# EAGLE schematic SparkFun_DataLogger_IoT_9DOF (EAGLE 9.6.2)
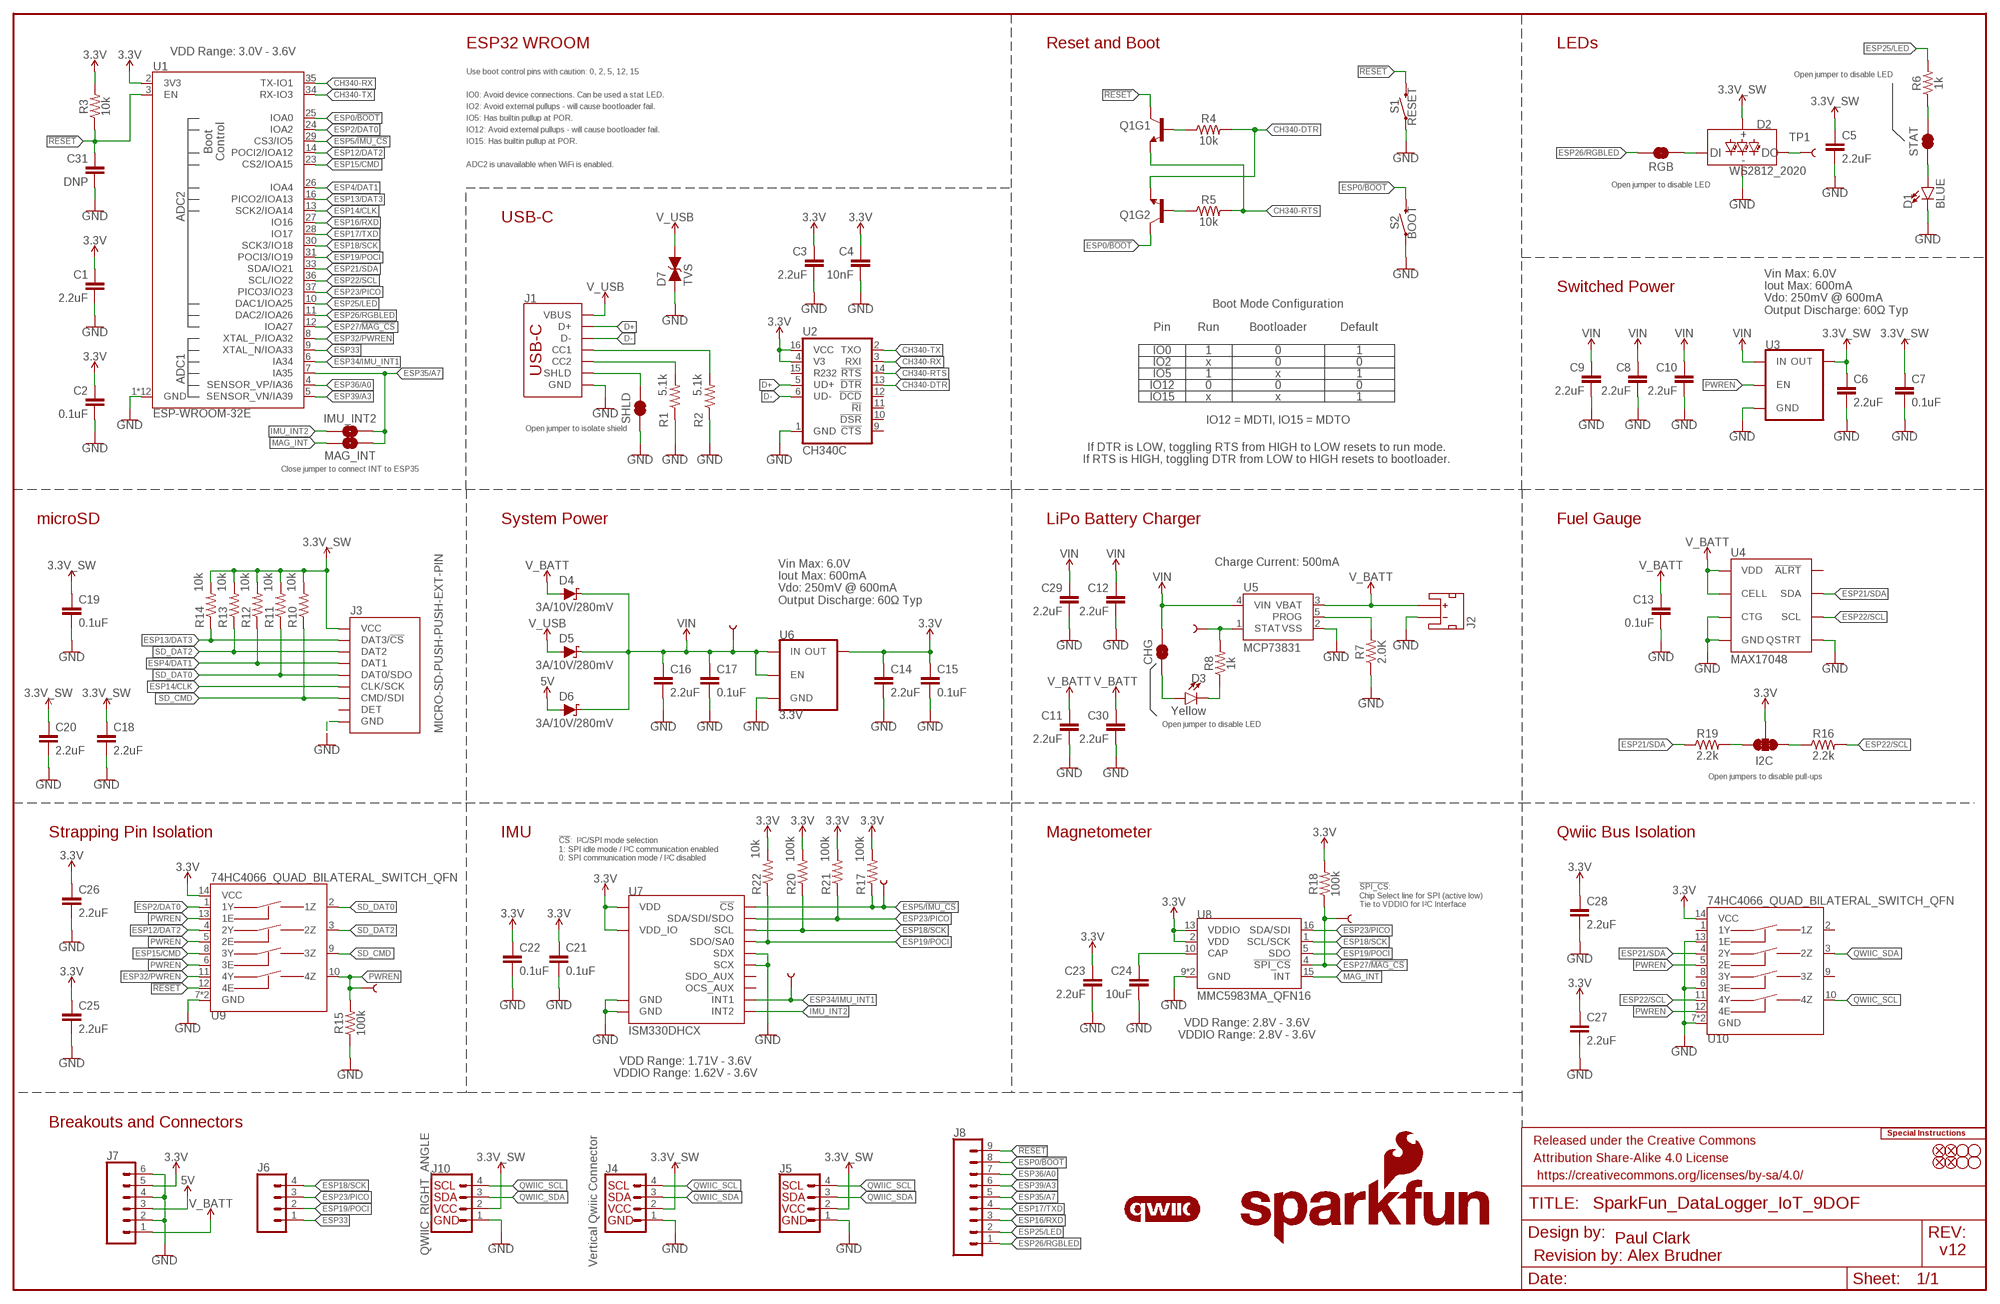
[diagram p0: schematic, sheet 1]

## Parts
C1  2.2uF  2.2UF-0402_TIGHT-10V-10%-X5R  [0402-TIGHT]
C2  0.1uF  0.1UF-0402T-6.3V-10%-X7R  [0402-TIGHT]
C3  2.2uF  2.2UF-0402_TIGHT-10V-10%-X5R  [0402-TIGHT]
C4  10nF  10NF-0402T-25V-10%-X7R-WE  [0402-TIGHT]
C5  2.2uF  2.2UF-0402_TIGHT-10V-10%-X5R  [0402-TIGHT]
C6  2.2uF  2.2UF-0402_TIGHT-10V-10%-X5R  [0402-TIGHT]
C7  0.1uF  0.1UF-0402T-6.3V-10%-X7R  [0402-TIGHT]
C8  2.2uF  2.2UF-0402_TIGHT-10V-10%-X5R  [0402-TIGHT]
C9  2.2uF  2.2UF-0402_TIGHT-10V-10%-X5R  [0402-TIGHT]
C10  2.2uF  2.2UF-0402_TIGHT-10V-10%-X5R  [0402-TIGHT]
C11  2.2uF  2.2UF-0402_TIGHT-10V-10%-X5R  [0402-TIGHT]
C12  2.2uF  2.2UF-0402_TIGHT-10V-10%-X5R  [0402-TIGHT]
C13  0.1uF  0.1UF-0402T-6.3V-10%-X7R  [0402-TIGHT]
C14  2.2uF  2.2UF-0402_TIGHT-10V-10%-X5R  [0402-TIGHT]
C15  0.1uF  0.1UF-0402T-6.3V-10%-X7R  [0402-TIGHT]
C16  2.2uF  2.2UF-0402_TIGHT-10V-10%-X5R  [0402-TIGHT]
C17  0.1uF  0.1UF-0402T-6.3V-10%-X7R  [0402-TIGHT]
C18  2.2uF  2.2UF-0402_TIGHT-10V-10%-X5R  [0402-TIGHT]
C19  0.1uF  0.1UF-0402T-6.3V-10%-X7R  [0402-TIGHT]
C20  2.2uF  2.2UF-0402_TIGHT-10V-10%-X5R  [0402-TIGHT]
C21  0.1uF  0.1UF-0402T-6.3V-10%-X7R  [0402-TIGHT]
C22  0.1uF  0.1UF-0402T-6.3V-10%-X7R  [0402-TIGHT]
C23  2.2uF  2.2UF-0402_TIGHT-10V-10%-X5R  [0402-TIGHT]
C24  10uF  10UF-0402T-6.3V-20%  [0402-TIGHT]
C25  2.2uF  2.2UF-0402_TIGHT-10V-10%-X5R  [0402-TIGHT]
C26  2.2uF  2.2UF-0402_TIGHT-10V-10%-X5R  [0402-TIGHT]
C27  2.2uF  2.2UF-0402_TIGHT-10V-10%-X5R  [0402-TIGHT]
C28  2.2uF  2.2UF-0402_TIGHT-10V-10%-X5R  [0402-TIGHT]
C29  2.2uF  2.2UF-0402_TIGHT-10V-10%-X5R  [0402-TIGHT]
C30  2.2uF  2.2UF-0402_TIGHT-10V-10%-X5R  [0402-TIGHT]
C31  DNP  DNP-0402-TIGHT_NO_CREAM  [0402-TIGHT_NO_CREAM]
CHG  JUMPER-SMT_2_NC_TRACE_SILK  [SMT-JUMPER_2_NC_TRACE_SILK]
D1  BLUE  LED-BLUE0603  [LED-0603]
D2  WS2812_2020  [WS2812-2020]
D3  Yellow  LED-YELLOW0603  [LED-0603]
D4  3A/10V/280mV  DIODE-SCHOTTKY-BAT60A  [SOD-323]
D5  3A/10V/280mV  DIODE-SCHOTTKY-BAT60A  [SOD-323]
D6  3A/10V/280mV  DIODE-SCHOTTKY-BAT60A  [SOD-323]
D7  TVS  DIODE_TVS  [0603]
FD1  FIDUCIAL1X2  [FIDUCIAL-1X2]
FD2  FIDUCIAL1X2  [FIDUCIAL-1X2]
FD3  FIDUCIAL1X2  [FIDUCIAL-1X2]
FD4  FIDUCIAL1X2  [FIDUCIAL-1X2]
FRAME1  FRAME-LEDGER  [CREATIVE_COMMONS]
H1  STAND-OFFTIGHT  [STAND-OFF-TIGHT]
H2  STAND-OFFTIGHT  [STAND-OFF-TIGHT]
H3  STAND-OFFTIGHT  [STAND-OFF-TIGHT]
H4  STAND-OFFTIGHT  [STAND-OFF-TIGHT]
I2C  JUMPER-SMT_3_2-NC_TRACE_SILK  [SMT-JUMPER_3_2-NC_TRACE_SILK]
IMU_!CS!  TEST-POINT3X5  [PAD.03X.05]
IMU_INT1  TEST-POINT3X5  [PAD.03X.05]
IMU_INT2  JUMPER-SMT_2_NO_SILK  [SMT-JUMPER_2_NO_SILK]
J1  USB_C_4-LAYER_PADS  [USB-C-16P_4LAYER-PADS]
J2  JST_2MM_MALE  [JST-2-SMD]
J3  MICRO-SD-PUSH-PUSH-EXT-PIN  [MICROSD-EXTERNALPIN]
J4  Vertical Qwiic Connector  QWIIC_CONNECTOR  [JST04_1MM_VERT]
J5  I2C_STANDARD_NO_SILK  [1X04_NO_SILK]
J6  CONN_041X04_NO_SILK_NO_POP  [1X04_NO_SILK]
J7  CONN_06NO_SILK_NO_POP  [1X06_NO_SILK]
J8  CONN_09NO_SILK  [1X09_NO_SILK]
J10  QWIIC_RIGHT_ANGLE  QWIIC_CONNECTORJS-1MM  [JST04_1MM_RA]
LOGO1  SPECIAL_INSTRUCTIONS-ORDERING  [ORDERING_INSTRUCTIONS]
LOGO3  QWIIC_LOGO_6MM  [QWIIC_6MM]
LOGO5  SFE_LOGO_NAME.2_INCH  [SFE_LOGO_NAME_.2]
LOGO6  SFE_LOGO_FLAME.2_INCH  [SFE_LOGO_FLAME_.2]
MAG_!CS!  TEST-POINT3X5  [PAD.03X.05]
MAG_INT  JUMPER-SMT_2_NO_SILK  [SMT-JUMPER_2_NO_SILK]
PWREN  TEST-POINT3X5  [PAD.03X.05]
Q1  TRANS_NPN_DUAL-MBT3904DW1T1  [SC70-6]
R1  5.1k  5.1KOHM-0402T-1/16W-1%  [0402-TIGHT]
R2  5.1k  5.1KOHM-0402T-1/16W-1%  [0402-TIGHT]
R3  10k  10KOHM-0402T-1/16W-1%  [0402-TIGHT]
R4  10k  10KOHM-0402T-1/16W-1%  [0402-TIGHT]
R5  10k  10KOHM-0402T-1/16W-1%  [0402-TIGHT]
R6  1k  1KOHM-0402T-1/16W-1%  [0402-TIGHT]
R7  2.0K  2.0KOHM-0402T-1/16W-1%  [0402-TIGHT]
R8  1k  1KOHM-0402T-1/16W-1%  [0402-TIGHT]
R10  10k  10KOHM-0402T-1/16W-1%  [0402-TIGHT]
R11  10k  10KOHM-0402T-1/16W-1%  [0402-TIGHT]
R12  10k  10KOHM-0402T-1/16W-1%  [0402-TIGHT]
R13  10k  10KOHM-0402T-1/16W-1%  [0402-TIGHT]
R14  10k  10KOHM-0402T-1/16W-1%  [0402-TIGHT]
R15  100k  100KOHM-0402T-1/16W-1%  [0402-TIGHT]
R16  2.2k  2.2KOHM-0402T-1/16W-1%  [0402-TIGHT]
R17  100k  100KOHM-0402T-1/16W-1%  [0402-TIGHT]
R18  100k  100KOHM-0402T-1/16W-1%  [0402-TIGHT]
R19  2.2k  2.2KOHM-0402T-1/16W-1%  [0402-TIGHT]
R20  100k  100KOHM-0402T-1/16W-1%  [0402-TIGHT]
R21  100k  100KOHM-0402T-1/16W-1%  [0402-TIGHT]
R22  10k  10KOHM-0402T-1/16W-1%  [0402-TIGHT]
RGB  JUMPER-SMT_2_NC_TRACE_SILK  [SMT-JUMPER_2_NC_TRACE_SILK]
S1  RESET  MOMENTARY-SWITCH-SPST-SMD-RIGHT-ANGLE  [TACTILE_SWITCH_SMD_RIGHT_ANGLE]
S2  BOOT  MOMENTARY-SWITCH-SPST-SMD-RIGHT-ANGLE  [TACTILE_SWITCH_SMD_RIGHT_ANGLE]
SHLD  JUMPER-SMT_2_NC_TRACE_SILK  [SMT-JUMPER_2_NC_TRACE_SILK]
STAT  JUMPER-SMT_2_NC_TRACE_SILK  [SMT-JUMPER_2_NC_TRACE_SILK]
TP1  TEST-POINT3X5  [PAD.03X.05]
U1  ESP-WROOM-32E  ESP-WROOM-3232D-NARROW  [ESP-WROOM-32D-NARROW]
U2  CH340C  [SO016]
U3  3.3V  V_REG_AP2112K-3.3V  [SOT23-5]
U4  MAX17048  MAX17048DFN8  [DFN-8]
U5  MCP73831  [SOT23-5]
U6  3.3V  V_REG_AP2112K-3.3V  [SOT23-5]
U7  ISM330DHCX  [LGA-14L]
U8  MMC5983MA_QFN16  [LGA-16-3X3MM-4X4PINS]
U9  74HC4066_QUAD_BILATERAL_SWITCH_QFN  [14-QFN]
U10  74HC4066_QUAD_BILATERAL_SWITCH_QFN  [14-QFN]
VIN  TEST-POINT3X5  [PAD.03X.05]
VIN1  TEST-POINT3X5  [PAD.03X.05]

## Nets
3.3V: C1.1 C2.1 C3.1 C4.1 C14.1 C15.1 C21.1 C22.1 C23.1 C25.1 C26.1 C27.1 C28.1 I2C.2 J7.5 R3.2 R17.2 R18.2 R20.2 R21.2 R22.2 U1.2(3V3) U2.4(V3) U2.16(VCC) U6.5(OUT) U7.P5(VDD_IO) U7.P8(VDD) U8.2(VDD) U8.13(VDDIO) U9.14(VCC) U10.14(VCC)
3.3V_SW: C5.1 C6.1 C7.1 C18.1 C19.1 C20.1 D2.VCC J3.4(VCC) J4.2 J5.2 J10.2 R10.2 R11.2 R12.2 R13.2 R14.2 U3.5(OUT)
5V: D6.A J7.3
!RESET!: C31.1 J8.9 Q1.3(C) R3.1 S1.2 U1.3(EN) U9.12(4E)
CAP: C24.1 U8.10(CAP)
CH340-DTR: Q1.1(E) R4.2 U2.13(!DTR)
CH340-RTS: Q1.4(E) R5.2 U2.14(!RTS)
CH340-RX: U1.35(TX-IO1) U2.3(RXI)
CH340-TX: U1.34(RX-IO3) U2.2(TXO)
D+: J1.A6(D+) J1.B6(D+) U2.5(UD+)
D-: J1.A7(D-) J1.B7(D-) U2.6(UD-)
ESP0/!BOOT!: J8.8 Q1.6(C) S2.2 U1.25(IOA0)
ESP2/DAT0: U1.24(IOA2) U9.1(1Y)
ESP4/DAT1: J3.8(DAT1) R12.1 U1.26(IOA4)
ESP5/!IMU_CS!: IMU_!CS!.1 R17.1 U1.29(CS3/IO5) U7.P12(!CS!)
ESP12/DAT2: U1.14(POCI2/IOA12) U9.4(2Y)
ESP13/DAT3: J3.2(DAT3/!CS!) R14.1 U1.16(PICO2/IOA13)
ESP14/CLK: J3.5(CLK/SCK) U1.13(SCK2/IOA14)
ESP15/CMD: U1.23(CS2/IOA15) U9.8(3Y)
ESP16/RXD: J8.3 U1.27(IO16)
ESP17/TXD: J8.4 U1.28(IO17)
ESP18/SCK: J6.4 R20.1 U1.30(SCK3/IO18) U7.P13(SCL) U8.1(SCL/SCK)
ESP19/POCI: J6.2 R22.1 U1.31(POCI3/IO19) U7.P1(SDO/SA0) U8.5(SDO)
ESP21/SDA: R19.1 U1.33(SDA/IO21) U4.8(SDA) U10.4(2Y)
ESP22/SCL: R16.2 U1.36(SCL/IO22) U4.7(SCL) U10.11(4Y)
ESP23/PICO: J6.3 R21.1 U1.37(PICO3/IO23) U7.P14(SDA/SDI/SDO) U8.16(SDA/SDI)
ESP25/LED: J8.2 R6.2 U1.10(DAC1/IOA25)
ESP26/RGBLED: J8.1 RGB.2 U1.11(DAC2/IOA26)
ESP27/!MAG_CS!: MAG_!CS!.1 R18.1 U1.12(IOA27) U8.4(!SPI_CS!)
ESP32/PWREN: U1.8(XTAL_P/IOA32) U9.11(4Y)
ESP33: J6.1 U1.9(XTAL_N/IOA33)
ESP34/IMU_INT1: IMU_INT1.1 U1.6(IA34) U7.P4(INT1)
ESP35/A7: IMU_INT2.2 J8.5 MAG_INT.2 U1.7(IA35)
ESP36/A0: J8.7 U1.4(SENSOR_VP/IA36)
ESP39/A3: J8.6 U1.5(SENSOR_VN/IA39)
GND: C1.2 C2.2 C3.2 C4.2 C5.2 C6.2 C7.2 C8.2 C9.2 C10.2 C11.2 C12.2 C13.2 C14.2 C15.2 C16.2 C17.2 C18.2 C19.2 C20.2 C21.2 C22.2 C23.2 C24.2 C25.2 C26.2 C27.2 C28.2 C29.2 C30.2 C31.2 D1.C D2.GND D7.1(A) J1.GND J1.GND2(GND) J2.1(-) J3.6(GND) J3.10(GND) J3.11(GND) J3.12(GND) J3.13(GND) J4.1 J5.1 J7.2 J7.4 J7.6 J10.1 R1.1 R2.1 R7.1 R15.1 S1.1 S2.1 SHLD.1 U1.1(GND) U1.15(GND) U1.38(GND) U1.GND1(GND) U1.GNDT1(GND) U1.GNDT2(GND) U1.GNDT3(GND) U1.GNDT4(GND) U1.GNDT5(GND) U1.GNDT6(GND) U1.GNDT7(GND) U1.GNDT8(GND) U2.1(GND) U3.2(GND) U4.1(CTG) U4.4(GND) U4.6(QSTRT) U4.9(GND) U5.2(VSS) U6.2(GND) U7.P2(SDX) U7.P3(SCX) U7.P6(GND) U7.P7(GND) U8.9(GND) U8.11(GND) U9.7(GND) U9.EPAD(GND) U10.6(3E) U10.7(GND) U10.13(1E) U10.EPAD(GND)
IMU_INT2: IMU_INT2.1 U7.P9(INT2)
MAG_INT: MAG_INT.1 U8.15(INT)
N$1: J1.B5(CC2) R1.2
N$2: J1.A5(CC1) R2.2
N$4: Q1.2(B) R5.1
N$5: Q1.5(B) R4.1
N$6: R6.1 STAT.2
N$7: D2.DO TP1.1
N$8: CHG.1 D3.A
N$9: D3.C R8.1
N$10: R8.2 U5.1(STAT) VIN1.1
N$11: R7.2 U5.5(PROG)
N$12: D2.DI RGB.1
N$13: D1.A STAT.1
N$16: I2C.1 R16.1
N$17: I2C.3 R19.2
PWREN: PWREN.1 R15.2 U3.3(EN) U9.5(2E) U9.6(3E) U9.10(4Z) U9.13(1E) U10.5(2E) U10.12(4E)
QWIIC_SCL: J4.4 J5.4 J10.4 U10.10(4Z)
QWIIC_SDA: J4.3 J5.3 J10.3 U10.3(2Z)
SD_CMD: J3.3(CMD/SDI) R10.1 U9.9(3Z)
SD_DAT0: J3.7(DAT0/SDO) R11.1 U9.2(1Z)
SD_DAT2: J3.1(DAT2) R13.1 U9.3(2Z)
SHIELD: J1.SHLD1(SHLD) J1.SHLD2(SHLD) J1.SHLD3(SHLD) J1.SHLD4(SHLD) SHLD.2
V_BATT: C11.1 C13.1 C30.1 D4.A J2.2(+) J7.1 U4.2(CELL) U4.3(VDD) U5.3(VBAT)
V_USB: D5.A D7.2(C) J1.VBUS1(VBUS) J1.VBUS2(VBUS)
VIN: C8.1 C9.1 C10.1 C12.1 C16.1 C17.1 C29.1 CHG.2 D4.C D5.C D6.C U3.1(IN) U5.4(VIN) U6.1(IN) U6.3(EN) VIN.1
Unconnected: J2.NC1(PAD1) J2.NC2(PAD2) J3.9(DET) U2.9(!CTS) U2.10(!DSR) U2.11(!RI) U2.12(!DCD) U2.15(R232) U4.5(!ALRT) U7.P10(OCS_AUX) U7.P11(SDO_AUX) U10.1(1Y) U10.2(1Z) U10.8(3Y) U10.9(3Z)

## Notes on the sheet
- VDD Range: 3.0V - 3.6V | ESP32 WROOM | Reset and Boot | LEDs
- Use boot control pins with caution: 0, 2, 5, 12, 15
- Open jumper to disable LED
- IO0: Avoid device connections. Can be used a stat LED.
- IO2: Avoid external pullups - will cause bootloader fail.
- IO5: Has builtin pullup at POR.
- IO12: Avoid external pullups - will cause bootloader fail.
- IO15: Has builtin pullup at POR.
- ADC2 is unavailable when WiFi is enabled.
- Open jumper to disable LED
- USB-C
- Switched Power
- Boot Mode Configuration
- Vin Max: 6.0V
  Iout Max: 600mA
  Vdo: 250mV @ 600mA
  Output Discharge: 60Ω Typ
- Pin | Run | Bootloader | Default
- IO0 | 1 | 0 | 1
- IO2 | x | 0 | 0
- IO5 | 1 | x | 1
- IO12 | 0 | 0 | 0
- IO15 | x | x | 1
- IO12 = MDTI, IO15 = MDTO
- Open jumper to isolate shield
- If DTR is LOW, toggling RTS from HIGH to LOW resets to run mode.
  If RTS is HIGH, toggling DTR from LOW to HIGH resets to bootloader.
- Close jumper to connect INT to ESP35
- microSD | System Power | LiPo Battery Charger | Fuel Gauge
- Charge Current: 500mA
- Vin Max: 6.0V
  Iout Max: 600mA
  Vdo: 250mV @ 600mA
  Output Discharge: 60Ω Typ
- Open jumper to disable LED
- Open jumpers to disable pull-ups
- Strapping Pin Isolation | IMU | Magnetometer | Qwiic Bus Isolation
- !CS!:  I²C/SPI mode selection
  1: SPI idle mode / I²C communication enabled
  0: SPI communication mode / I²C disabled
- !SPI_CS!:
  Chip Select line for SPI (active low) 
  Tie to VDDIO for I²C Interface
- VDD Range: 2.8V - 3.6V
  VDDIO Range: 2.8V - 3.6V
- VDD Range: 1.71V - 3.6V
  VDDIO Range: 1.62V - 3.6V
- Breakouts and Connectors
- Paul Clark
- v12
- Revision by: Alex Brudner

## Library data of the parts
C1 C3 C5 C6 C8-C12 C14 C16 C18 C20 C23 C25-C30 = SparkFun-Capacitors:2.2UF: 2.2µF ceramic capacitors; PROD_ID: CAP-14232
C2 C7 C13 C15 C17 C19 C21 C22 = SparkFun-Capacitors:0.1UF: 0.1µF ceramic capacitors; PROD_ID: CAP-14993
C4 = SparkFun-Capacitors:10NF: 0.01uF/10nF/10,000pF ceramic capacitors; PROD_ID: CAP-16508
C24 = SparkFun-Capacitors:10UF: 10.0µF ceramic capacitors; PROD_ID: CAP-14848
C31 = SparkFun-Capacitors:DNP: Do-Not-Populate capacitor
CHG RGB SHLD STAT = SparkFun-Jumpers:JUMPER-SMT_2_NC_TRACE: Normally closed trace jumper
D1 = SparkFun-LED:LED-BLUE: Blue SMD LED; PROD_ID: DIO-08575
D2 = SparkFun-LED:WS2812: Addressable RGB LED - 1 Wire Common names: WS2812, SK6812, Neopixel, APA-106, etc. SMD LED with built-in controller IC. Color: Red/Green/Blue SparkFun Products: LED-SMD RGB (WS2812) LED - RGB Addressable, PTH, 5mm Diffused (5 Pack) LED - RGB Addressable, PTH, 5mm Clear (5 Pack) Blynk Board -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; PROD_ID: DIO-15591
D3 = SparkFun-LED:LED-YELLOW: Yellow SMD LED; PROD_ID: DIO-09003
D4-D6 = SparkFun-DiscreteSemi:DIODE-SCHOTTKY: Schottky diode; PROD_ID: DIO-14072
D7 = SparkFun-DiscreteSemi:DIODE_TVS; PROD_ID: DIO-14502; VALUE: 24V
FD1-FD4 = SparkFun-Aesthetics:FIDUCIAL: Fiducial Alignment Points
FRAME1 = SparkFun-Aesthetics:FRAME-LEDGER: Schematic Frame - Ledger
H1-H4 = SparkFun-Hardware:STAND-OFF: Stand Off
I2C = SparkFun-Jumpers:JUMPER-SMT_3_2-NC_TRACE: Normally closed trace jumper (2 of 2 connections) This jumper has a trace between all three pads so they are normally closed (NC). Use a razor knife to open the connection(s). For best results follow the IPC guidelines for cutting traces: Cutout at least 0.063 mm (0.005 in). Remove all loose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
IMU_!CS! IMU_INT1 MAG_!CS! PWREN TP1 VIN VIN1 = SparkFun-Connectors:TEST-POINT: SparkFun Test Points
IMU_INT2 MAG_INT = SparkFun-Jumpers:JUMPER-SMT_2_NO: Normally open jumper
J1 = SparkFun-Connectors:USB_C: USB Type C 16Pin Connector Super Speed pins not available on the 16-pin purely SMD connector so this part is best for USB 2.0 implementations. D1 and D2 are tied together enabling D+/- no matter which way the cable is plugged into the connector. The two channel configuration pins (CC1/2) are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; PROD_ID: CONN-14122
J2 = SparkFun-Connectors:JST_2MM_MALE: JST 2MM MALE RA CONNECTOR Two pin, compact surface mount connector. Commonly used as a battery input connection point. We really like the solid locking feeling and high current rating on these small connectors. We use these all the time as battery connectors. Mates to single-cell LiPo batteries.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; PROD_ID: CONN-11443; SF_ID: PRT-08612
J3 = SparkFun-Connectors:MICRO-SD: microSD Socket for Transflash Various sockets for µSD. tDoc lines correctly indicate media card edge positions when inserting (unlocked, locked, depressed). NOTE: CD1 and CD2 are connected internally, and the default detect state of the socket is detect pin to ground. SparkFun Products: WAV Trigger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; PROD_ID: CONN-16110
J4 = SparkFun-Connectors:QWIIC_CONNECTOR: SparkFun I2C Standard Qwiic Connector An SMD 1mm pitch JST connector makes it easy and quick (get it? Qwiic?) to connect I2C devices to each other. The Qwiic system enables fast and solderless connection between popular platforms and various sensors and actuators. We carry 200mm, 100mm, 50mm, and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; PROD_ID: CONN-14483
J5 = SparkFun-Connectors:I2C_STANDARD: SparkFun I2C Standard Pinout Header SparkFun has standardized on a pinout for all I2C based sensor breakouts. This pinout allows I2C boards to be plugged directly into the headers on Arduino Uno compatible boards, and to be daisy chained easily. Example SparkFun Products: SparkFun Atmospheric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
J6 = SparkFun-Connectors:CONN_04: Multi connection point. Often used as Generic Header-pin footprint for 0.1 inch spaced/style header connections On any of the 0.1 inch spaced packages, you can populate with these: Break Away Headers - Straight (PRT-00116) Break Away Male Headers - Right Angle (PRT-00553) Female Headers (PRT-00115)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
J7 = SparkFun-Connectors:CONN_06: Multi connection point. Often used as Generic Header-pin footprint for 0.1 inch spaced/style header connections On any of the 0.1 inch spaced packages, you can populate with these: Break Away Headers - Straight (PRT-00116) Break Away Male Headers - Right Angle (PRT-00553) Female Headers (PRT-00115)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
J8 = SparkFun-Connectors:CONN_09: Multi connection point. Often used as Generic Header-pin footprint for 0.1 inch spaced/style header connections On any of the 0.1 inch spaced packages, you can populate with these: Break Away Headers - Straight (PRT-00116) Break Away Male Headers - Right Angle (PRT-00553) Female Headers (PRT-00115)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
J10 = SparkFun-Connectors:QWIIC_CONNECTOR: SparkFun I2C Standard Qwiic Connector An SMD 1mm pitch JST connector makes it easy and quick (get it? Qwiic?) to connect I2C devices to each other. The Qwiic system enables fast and solderless connection between popular platforms and various sensors and actuators. We carry 200mm, 100mm, 50mm, and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; PROD_ID: CONN-13694
LOGO1 = SparkFun-Aesthetics:SPECIAL_INSTRUCTIONS: Special Ordering/Production Instructions Alert
LOGO3 = SparkFun-Aesthetics:QWIIC_LOGO: Qwiic Logos for placement on schematic and PCB. The 5.5mm silk logo is best for placing next to Qwiic connector.
LOGO5 = SparkFun-Aesthetics:SFE_LOGO_NAME: SparkFun Font Logo
LOGO6 = SparkFun-Aesthetics:SFE_LOGO_FLAME: SparkFun Flame Logo
Q1 = SparkFun-DiscreteSemi:TRANS_NPN_DUAL: Dual NPN Transistors in Single Package The MBT3904W1 puts two general purpose 3904 NPN transistors in a single package. Datasheet SparkFun Products: SparkFun ESP32 Thing; PROD_ID: TRANS-13337
R1 R2 = SparkFun-Resistors:5.1KOHM; PROD_ID: RES-14340
R3-R5 R10-R14 R22 = SparkFun-Resistors:10KOHM: 10kΩ resistor; PROD_ID: RES-14241
R6 R8 = SparkFun-Resistors:1KOHM: 1kΩ resistor; PROD_ID: RES-14342
R7 = SparkFun-Resistors:2.0KOHM: 2kΩ resistor; PROD_ID: RES-15406
R15 R17 R18 R20 R21 = SparkFun-Resistors:100KOHM: 100kΩ resistor; PROD_ID: RES-13495
R16 R19 = SparkFun-Resistors:2.2KOHM: 2.2kΩ resistor; PROD_ID: RES-14341
S1 S2 = SparkFun-Switches:MOMENTARY-SWITCH-SPST: Momentary Switch (Pushbutton) - SPST; PROD_ID: COMP-12265
U1 = SparkFun-RF:ESP-WROOM-32: ESP-WROOM-32D - trace antenna (includes keepout) ESP-WROOM-32U - U.FL antenna connector Includes both "standard" footprints and "narrow" version (for use with tighter layouts).; PROD_ID: IC-15676
U2 = SparkFun-IC-Comms:CH340C; PROD_ID: IC-14038
U3 U6 = SparkFun-IC-Power:V_REG_AP2112: AP2112 - 600mA CMOS LDO Regulator w/ Enable The AP2112 is CMOS process low dropout linear regulator with enable function, the regulator delivers a guaranteed 600mA (min.) continuous load current. Features Output Voltage Accuracy: ±1.5% Output Current: 600mA (Min.) Foldback Short Current Protection: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; PROD_ID: VREG-12457
U4 = SparkFun-IC-Power:MAX17048: Micropower 1-Cell Li+ ModelGauge SparkFun Products Qduino Mini (DEV-13614); PROD_ID: IC-12551
U5 = SparkFun-IC-Power:MCP73831: MCP73831T Li-Ion, Li-Pol Controller Miniature single cell, fully integrated Li-Ion, Li-polymer charge management controller Datasheet SparkFun Products: SparkFun ESP32 Thing SparkFun 9DoF Razor IMU M0; PROD_ID: IC-09995
U7 = SparkFun-Sensors:ISM330DHCX: ISM330DHCX 6DoF The ISM330DHCX is a system-in-package featuring a high-performance 3D digital accelerometer and 3D digital gyroscope tailored for Industry 4.0 applications.; PROD_ID: IC-16693
U8 = SparkFun-Sensors:MMC5983MA: High Performance 3-axis Magnetic Sensor The MMC5983MA is an AEC-Q100 qualified complete 3-axis magnetic sensor with on-chip signal processing and integrated I2C/SPI bus suitable for use in automotive applications. The device can be connected directly to a microprocessor, eliminating the need for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; PROD_ID: IC-16314
U9 U10 = SparkFun-IC-Logic:74HC4066_QUAD_BILATERAL_SWITCH: Nexperia Quad Bilateral Switch The 74HC4066 is a quad single pole, single throw analog switch. Each switch features two input/output terminals (nY and nZ) and an active HIGH enable input (nE). When nE is LOW, the analog switch is turned off. Inputs include clamp diodes. This enables the use of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; PROD_ID: IC-16528

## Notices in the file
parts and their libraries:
SparkFun-Aesthetics: Licensing: Creative Commons ShareAlike 4.0 International - https://creativecommons.org/licenses/by-sa/4.0
SparkFun-Aesthetics: Released under the Creative Commons Attribution Share-Alike 4.0 License
SparkFun-Aesthetics: https://creativecommons.org/licenses/by-sa/4.0
